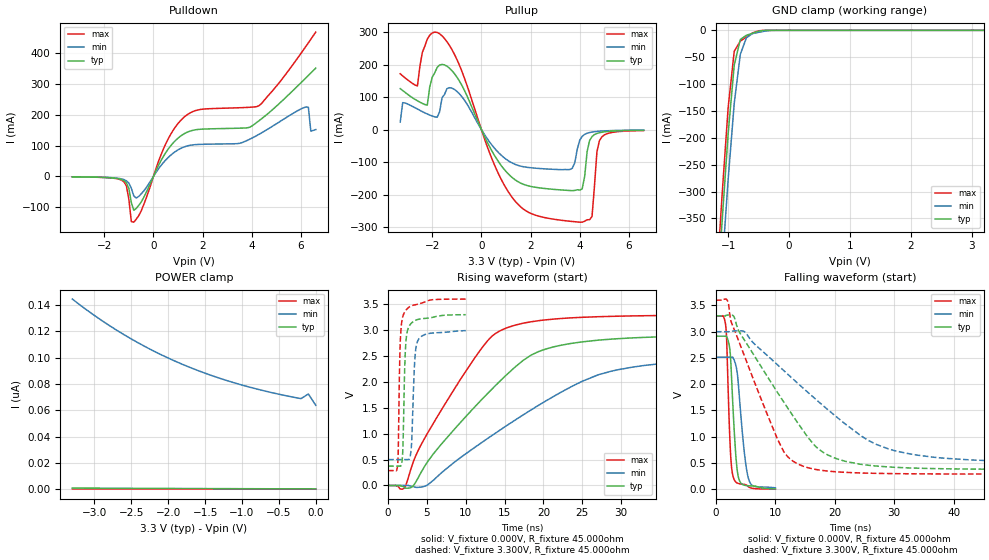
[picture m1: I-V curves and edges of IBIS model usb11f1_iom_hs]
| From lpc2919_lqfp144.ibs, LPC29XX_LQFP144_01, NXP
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| usb11f1
|   Universal Serial Bus Pad
|   Revision 1.1 Specification
|   Programmable Single Ended Core Input
|   Forced Single Ended Low
|   Switchable between
|   - high speed output mode
|   - low speed output mode
|   - low/high speed input mode
| |   Rev 0.20 IBIS Model Design Automation Generation   |
| |   N O N - S I L I C O N   C O R R E L A T E D   |
| |   This IBIS [Model] is pre-Beta tactical support   |
| |  Note: this IBIS [Model] contains clamp curves generated   |
| |   through simulation which should not be relied upon   |
| Pccmos14 hliolib_nlm 4.0
|   0.18 um 3.3V pad library
|   six level metal
|   dual oxide
|   single threshold voltage
|   nominal line mixed supply
|   parasitic extracted netlists
| Process block c14
| High Speed Output Mode
[Model]   usb11f1_iom_hs | of usb11f1
Model_type   I/O
Polarity   Non-Inverting
Enable   Active-Low
|  Reciever Thresholds
Vinl   = 0.8V
Vinh   = 2.0V
| AC Test Load Conditions
Vref   = 0
Cref   = 0
Rref   = 1000000000
Vmeas   = 1.65
| [Process Range]   typical   min   max
| C_comp edge width   400.000ps   400.000ps   400.000ps
| C_comp Tstrobe   40.000fs   40.000fs   40.000fs
C_comp   3.752pF   3.496pF   4.045pF
[Temperature Range]   25   125   -40
[Voltage Range]   3.30V   3.00V   3.60V
[GND Clamp Reference]   0.00V   0.00V   0.00V
[Pulldown Reference]   0.00V   0.00V   0.00V
[POWER Clamp Reference]   3.30V   3.00V   3.60V
[Pullup Reference]   3.30V   3.00V   3.60V
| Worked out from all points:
|   slope of the pulldown table from 0 to 0.495 V, typ, clamps not added: 6.48 ohm
|   slope of the pullup table from 0 to 0.495 V, typ, clamps not added: 6.61 ohm
|   GND clamp passes 1 mA (typ) near -0.46 V on its own axis
|   rising waveform, V_fixture 0.000V, R_fixture 45.000ohm: 20-80 % time 11ns typ, 15.9ns min, 8.17ns max; typ from 0 V to 2.91 V
|   falling waveform, V_fixture 0.000V, R_fixture 45.000ohm: 20-80 % time 845ps typ, 1.21ns min, 607ps max; typ from 2.91 V to 0.006 V
|   rising waveform, V_fixture 3.300V, R_fixture 45.000ohm: 20-80 % time 320ps typ, 399ps min, 287ps max; typ from 0.374 V to 3.3 V
|   falling waveform, V_fixture 3.300V, R_fixture 45.000ohm: 20-80 % time 10.2ns typ, 15.5ns min, 6.95ns max; typ from 3.3 V to 0.374 V
[GND Clamp]
| ref voltage   0.00V   0.00V   0.00V
|   Voltage   I(typ)   I(min)   I(max)
-3.3V     -4.618A    -4.67A     -4.591A
-1.2V     -533.4mA   -616mA     -486.2mA
-1.1V     -356.1mA   -441.1mA   -306.9mA
-1V       -192.1mA   -277.1mA   -143.8mA
-900mV    -64.59mA   -135.6mA   -38.91mA
-800mV    -17.04mA   -44.51mA   -19.95mA
-700mV    -9.237mA   -13.86mA   -12.52mA
-600mV    -5.456mA   -6.064mA   -4.789mA
-500mV    -1.495mA   -3.666mA   -840.2uA
-300mV    -6.625uA   -179.7uA   -408.9nA
3.2V      293.2pA    68.89nA    105.6pA
[Power Clamp]   | Vtable = Vcc - Vpad
| ref voltage   3.30V   3.00V   3.60V
|   Voltage   I(typ)   I(min)   I(max)
-3.3V     1.005nA    144.5nA    354.7pA
-3V       911.2pA    132nA      335.1pA
-2.6V     800.8pA    117.4nA    309pA
-2.3V     727.5pA    108nA      289.6pA
-1.9V     640.7pA    97.15nA    263.8pA
-1.6V     582.9pA    90.25nA    244.5pA
-1.3V     530.6pA    84.3nA     225.3pA
-1V       483pA      79.18nA    206.1pA
-700mV    439.6pA    74.79nA    187pA
-200mV    377.6pA    68.89nA    155pA
-100mV    416.5pA    72.39nA    142.6pA
0V        319.1pA    63.83nA    125.6pA
[Pulldown]
| ref voltage   0.00V   0.00V   0.00V
|   Voltage   I(typ)   I(min)   I(max)
-3.3V     -1.652mA   -1.454mA   -1.796mA
-1.2V     -13.92mA   -10.45mA   -17.73mA
-1.1V     -21.12mA   -14.45mA   -30.61mA
-900mV    -85.23mA   -38.63mA   -146.6mA
-800mV    -110mA     -63.62mA   -148.7mA
500mV     77.03mA    53.28mA    105.7mA
1.1V      130.5mA    90.36mA    180.9mA
4.3V      181mA      136.8mA    229.8mA
6.2V      319.7mA    225.1mA    421.9mA
6.3V      327.6mA    224.1mA    433.3mA
6.4V      335.5mA    146.8mA    444.9mA
6.6V      351.2mA    151.8mA    468.2mA
[Pullup]   | Vtable = Vcc - Vpad
| ref voltage   3.30V   3.00V   3.60V
|   Voltage   I(typ)   I(min)   I(max)
-3.3V     125.8mA    23.2mA     171.5mA
-2.6V     88.3mA     62.98mA    134mA
-2.2V     74.98mA    47.7mA     277.9mA
-1.6V     200.3mA    97.67mA    288.3mA
-1V       161.8mA    117.7mA    216.4mA
900mV     -120mA     -85.3mA    -166.8mA
2.5V      -180.9mA   -120.7mA   -269.8mA
3.7V      -188.1mA   -119.1mA   -283mA
4.1V      -182.9mA   -20.96mA   -285.2mA
4.4V      -34.22mA   -9.287mA   -277.5mA
4.8V      -9.883mA   -5.195mA   -34.66mA
6.6V      -2.365mA   -1.804mA   -3.161mA
[Ramp]
R_load   = 60.000ohm
|   dV/dt(typ)   dV/dt(min)   dV/dt(max)
dV/dt_r   803.394mV/4.105ns   370.492mV/2.885ns   1.331V/4.905ns
dV/dt_f   843.371mV/4.620ns   360.067mV/3.240ns   1.540V/5.255ns
[Rising Waveform]  | cubic spline decimation from 16001 points
V_fixture   = 0.000V
R_fixture   = 45.000ohm
|   Time   V(typ)   V(min)   V(max)
0s        443.9pV    34.48nV    250.2pV
2.05ns    -28.68mV   9.864uV    -55.51mV
3.165ns   -16.71mV   -18.22mV   419.1mV
5.14ns    468.7mV    16.86mV    1.024V
12.03ns   1.653V     825.1mV    2.643V
16.32ns   2.281V     1.258V     3.093V
21.57ns   2.684V     1.741V     3.215V
26.99ns   2.804V     2.132V     3.257V
32.92ns   2.858V     2.315V     3.276V
80ns      2.912V     2.506V     3.295V
[Falling Waveform]  | cubic spline decimation from 2001 points
V_fixture   = 0.000V
R_fixture   = 45.000ohm
|   Time   V(typ)   V(min)   V(max)
0s        2.914V     2.514V     3.296V
1.65ns    2.919V     2.514V     3.102V
1.79ns    2.905V     2.514V     2.86V
2.415ns   2.567V     2.514V     760.7mV
2.935ns   1.397V     2.492V     222.4mV
3.365ns   607.8mV    2.348V     134.4mV
3.78ns    227.5mV    1.985V     109.9mV
4.655ns   81.21mV    824.9mV    94.37mV
5.45ns    66.93mV    210.5mV    47.53mV
10ns      6.197mV    27.24mV    1.84mV
[Rising Waveform]  | cubic spline decimation from 2001 points
V_fixture   = 3.300V
V_fixture_min = 3.000V
V_fixture_max = 3.600V
R_fixture   = 45.000ohm
|   Time   V(typ)   V(min)   V(max)
0s        373.7mV    499.4mV    287.7mV
1.215ns   373.7mV    499.4mV    375.2mV
1.575ns   374.2mV    499.5mV    2.78V
1.87ns    595mV      499.5mV    3.244V
2.065ns   1.779V     499.5mV    3.327V
2.355ns   2.862V     499.5mV    3.393V
2.96ns    3.126V     677.4mV    3.465V
3.43ns    3.18V      2.396V     3.486V
3.84ns    3.205V     2.798V     3.499V
10ns      3.296V     2.989V     3.598V
[Falling Waveform]  | cubic spline decimation from 16001 points
V_fixture   = 3.300V
V_fixture_min = 3.000V
V_fixture_max = 3.600V
R_fixture   = 45.000ohm
|   Time   V(typ)   V(min)   V(max)
0s        3.3V       3V         3.6V
1.96ns    3.316V     3V         3.585V
2.955ns   3.297V     3.013V     3.074V
4.81ns    2.836V     3V         2.532V
11.41ns   1.661V     2.26V      717.5mV
14.73ns   1.108V     1.92V      436.6mV
20.49ns   574.7mV    1.36V      330.4mV
25.63ns   457.1mV    931.8mV    306.2mV
31.99ns   408.5mV    686.3mV    295.4mV
80ns      374.5mV    503.6mV    287.9mV
